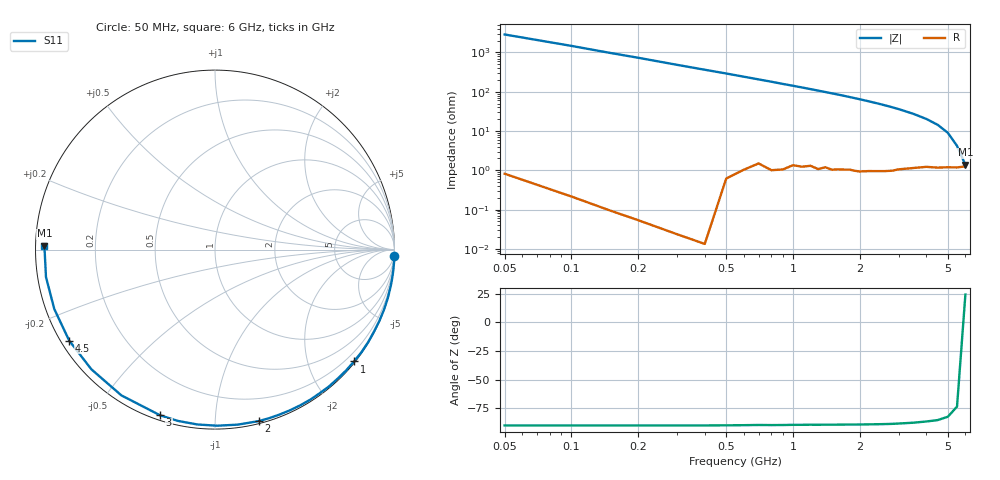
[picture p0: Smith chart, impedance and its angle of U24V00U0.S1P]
! SIEMENS Discrete & RF Semiconductors
! BBY52-02W
! Si Tuning Diode in SCD-80
! VR = 4 V
! S-Parameters:  September  1997
# GHz  S  MA  R  50
!  f  S11
! GHz  MAG  ANG
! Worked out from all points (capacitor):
!   34 points, 50 MHz to 6 GHz, reference 50 ohm
!   read as one part to ground: C = 1.09 pF near 50 MHz
!   lowest |Z| = 1.38 ohm at 6 GHz (marker M1)
!   series resonance near 5.938 GHz, so ESL is about 660 pH
!   S11 on the Smith chart (normalised r, x): 50 MHz: 0, -57; 1 GHz: 0.03, -2.84; 2 GHz: 0.02, -1.29; 3 GHz: 0.02, -0.72; 4.5 GHz: 0.02, -0.29; 6 GHz: 0.03, +0.01
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0.05  1 -2.0
0.2  1 -7.8
0.3  1 -11.8
0.4  1 -15.7
0.5  0.9993 -19.5
0.6  0.9983 -23.4
0.8  0.9971 -31.1
0.9  0.9962 -35.1
1  0.9941 -38.8
1.1  0.9935 -42.6
1.3  0.9923 -50.2
1.5  0.9904 -57.6
1.6  0.9891 -61.2
1.7  0.9881 -64.8
1.8  0.9869 -68.5
1.9  0.9866 -72.1
2  0.9861 -75.6
2.2  0.9835 -82.5
2.4  0.9813 -89.3
2.6  0.9792 -95.8
2.8  0.9766 -102.2
3  0.9726 -108.3
3.5  0.9653 -122.7
4  0.9587 -135.9
4.5  0.9576 -148.0
5  0.9547 -159.7
5.5  0.954 -170.8
6  0.9508 178.7
